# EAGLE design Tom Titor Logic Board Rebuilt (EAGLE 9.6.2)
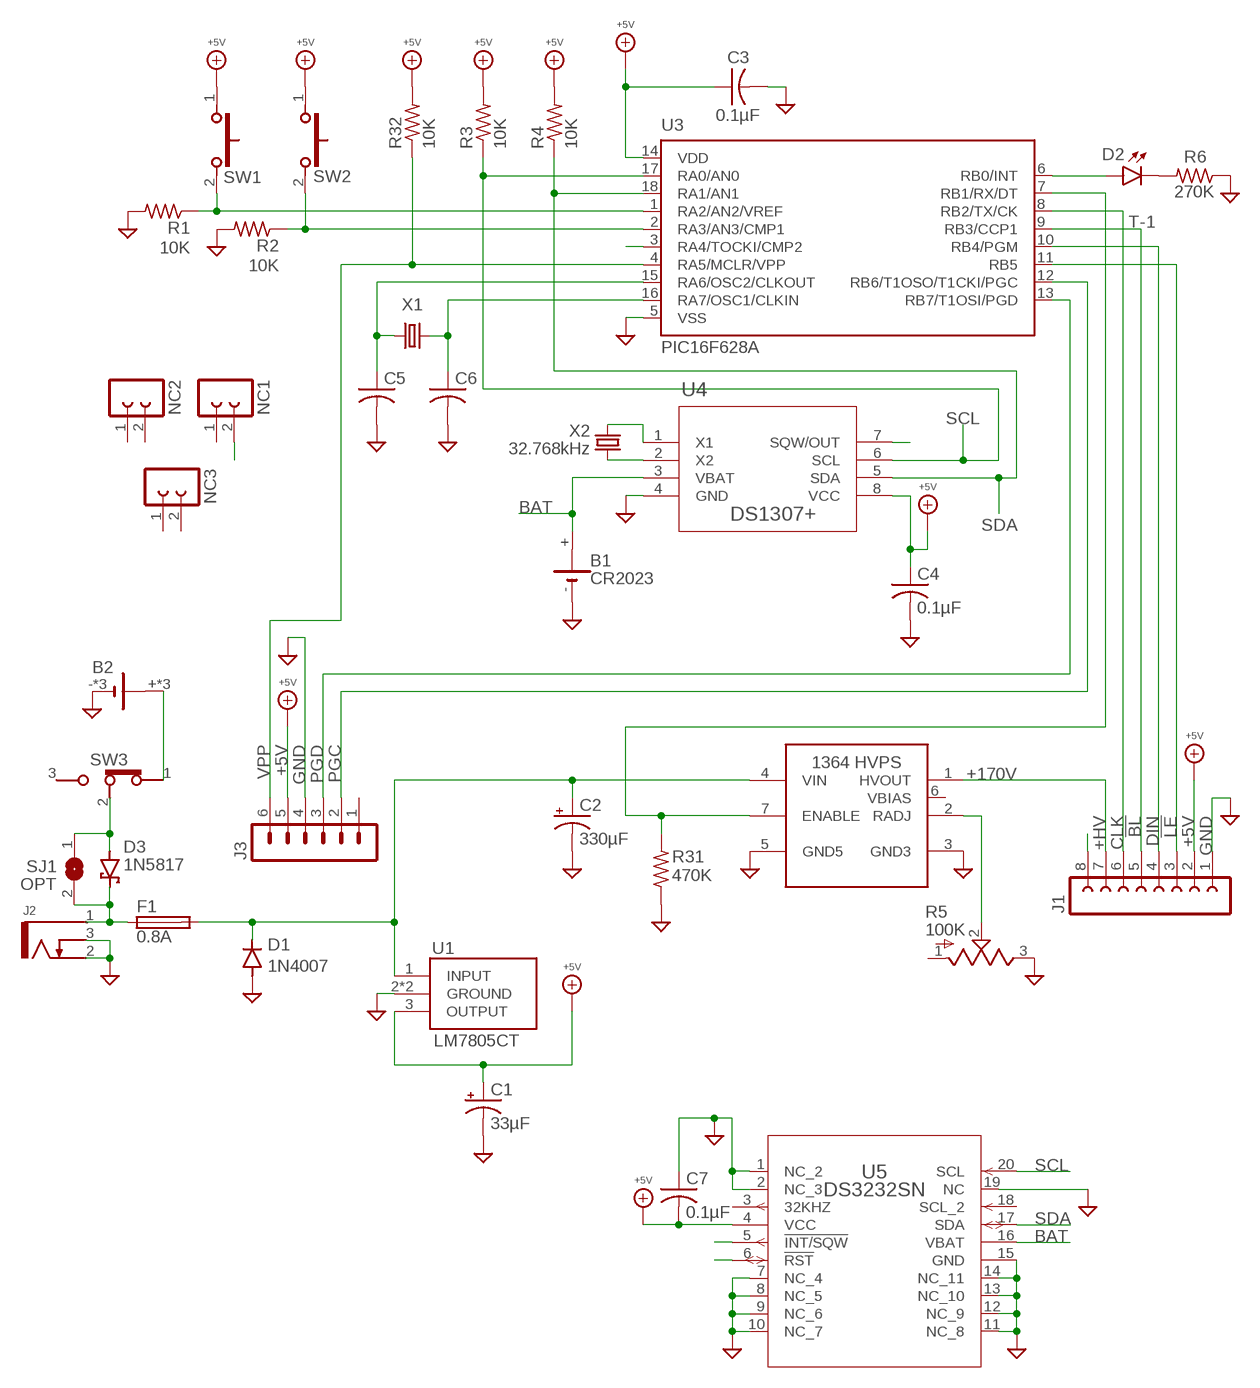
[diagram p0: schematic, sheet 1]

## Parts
B1  CR2023  BATTERY  [103]
B2  BATTERYWIRE_ATTACH  [BATTERY_WIRE]
C1  33µF  CPOL-USE2-5  [E2-5]
C2  330µF  CPOL-USE3.5-8  [E3,5-8]
C3  0.1µF  C-US  [C025-040X050]
C4  0.1µF  C-US  [C025-040X050]
C5  0.1µF  C-US  [C025-040X050]
C6  0.1µF  C-US  [C025-040X050]
C7  0.1µF  C-USC0805  [C0805]
D1  1N4007  RECTIFIER  [DO41-7]
D2  T-1  LED  [LED3MM]
D3  1N5817  SCHOTTKY  [DO41-7]
F1  0.8A  FUSE  [5X20MM]
J1  FE08  [FE08]
J2  KLDX-0202-B  [KDLX-0202-X]
J3  MA06  [MA06]
NC1  FE02  [FE02]
NC2  FE02  [FE02]
NC3  FE02  [FE02]
R1  10K  R-US0207/10  [0207/10]
R2  10K  R-US0207/10  [0207/10]
R3  10K  R-US0207/10  [0207/10]
R4  10K  R-US0207/10  [0207/10]
R5  100K  R-US_TRIM  [PV37W]
R6  270K  R-US0207/10  [0207/10]
R31  470K  R-US0207/10  [0207/10]
R32  10K  R-US0207/10  [0207/10]
SJ1  OPT  SJ  [SJ]
SW1  FSMRA4JH  SWITCH_PUSH_SPST_(ON)  [FSMRA4JH]
SW2  FSMRA4JH  SWITCH_PUSH_SPST_(ON)  [FSMRA4JH]
SW3  102-1261-EV  SWITCH_SLIDE_SPDT_ON  [SLIDE_SPDT_MINI]
U1  LM7805CT  MC7805CTG  [TO-220-3_RA]
U2  1364-HVPS-H  [1364-HVPS-H]
U3  PIC16F628A  PIC16F628P  [DIP-18]
U4  DS1307+  [DIP-8]
U5  DS3232SN  [SOIC-20]
X1  CRYSTAL  [HC18U-V_ALT]
X2  32.768kHz  CRYSTALTC38H  [TC38H]

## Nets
!BL!: J1.5 U3.9(RB3/CCP1)
!LE!: J1.3 U3.11(RB5)
+5V: C1.+ C3.1 C4.1 C7.2 J1.2 J3.5 R3.2 R4.2 R32.2 SW1.1 SW2.1 U1.3(OUTPUT) U3.14(VDD) U4.8(VCC) U5.4(VCC)
+9V: D3.C F1.1A F1.1B J2.1 SJ1.2
+9V_1: C2.+ D1.C F1.2A F1.2B U1.1(INPUT) U2.4(VIN)
+9V_2: D3.A SJ1.1 SW3.2(COM)
+9V_4: B2.+ B2.N$1(+) B2.N$2(+) SW3.1(POS_1)
+HV: J1.7 U2.1(HVOUT)
BAT: B1.+ U4.3(VBAT) U5.16(VBAT)
CLK: J1.6 U3.8(RB2/TX/CK)
DEBUG: D2.A D2.K(C) R6.2 U3.6(RB0/INT)
DIN: J1.4 U3.10(RB4/PGM)
ENABLE: R31.2 U2.7(ENABLE) U3.7(RB1/RX/DT)
GND: B1.- B2.- B2.N$3(-) B2.N$24(-) C1.- C2.- C3.2 C4.2 C5.2 C6.2 C7.1 D1.A J1.1 J2.2 J2.3 J3.4 R1.2 R2.2 R5.3 R6.1 R31.1 U1.2(GROUND) U1.2_1(GROUND) U2.3(GND3) U2.5(GND5) U3.5(VSS) U4.4(GND) U5.1(NC_2) U5.2(NC_3) U5.7(NC_4) U5.8(NC_5) U5.9(NC_6) U5.10(NC_7) U5.11(NC_8) U5.12(NC_9) U5.13(NC_10) U5.14(NC_11) U5.15(GND) U5.19(NC)
MYSTERY_1: J1.8
MYSTERY_2: U5.5(!INT/SQW)
MYSTERY_3: U5.6(!RST)
MYSTERY_4: U3.3(RA4/TOCKI/CMP2)
MYSTERY_5: U4.7(SQW/OUT)
N$1: U4.1(X1) X2.2
N$2: U4.2(X2) X2.1
N$5: NC1.2
PGC: J3.2 U3.12(RB6/T1OSO/T1CKI/PGC)
PGD: J3.3 U3.13(RB7/T1OSI/PGD)
RADJ: R5.2 U2.2(RADJ)
SCL: R3.1 U3.17(RA0/AN0) U4.6(SCL) U5.20(SCL)
SDA: R4.1 U3.18(RA1/AN1) U4.5(SDA) U5.17(SDA)
SUPP_CRYSTAL_1: C5.1 U3.15(RA6/OSC2/CLKOUT) X1.1
SUPP_CRYSTAL_2: C6.1 U3.16(RA7/OSC1/CLKIN) X1.2
SW1: R1.1 SW1.2 U3.1(RA2/AN2/VREF)
SW2: R2.1 SW2.2 U3.2(RA3/AN3/CMP1)
VPP: J3.6 R32.1 U3.4(RA5/MCLR/VPP)
Unconnected: J3.1 NC1.1 NC2.1 NC2.2 NC3.1 NC3.2 R5.1 SW3.3(POS_2) U2.6(VBIAS) U5.3(32KHZ) U5.18(SCL_2)

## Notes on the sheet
- +170V

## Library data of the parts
B1 B2 = My Imported Components:BATTERY: LI BATTERY Varta
C1 C2 = My Imported Components:CPOL-US
C3-C6 = My Imported Components:C-US
C7 = rcl:C-US: CAPACITOR, American symbol; SPICEPREFIX: C
D1 = My Imported Components:RECTIFIER
D2 = My Imported Components:LED
D3 = My Imported Components:SCHOTTKY
F1 = My Imported Components:FUSE
J1 = My Imported Components:FE08: FEMALE HEADER; OC_FARNELL: unknown; OC_NEWARK: unknown
J2 = My Imported Components:KLDX-0202-B: https://www.mouser.com/datasheet/2/222/KLDX_0202-334781.pdf
J3 = My Imported Components:MA06: PIN HEADER; OC_FARNELL: unknown; OC_NEWARK: unknown
NC1-NC3 = My Imported Components:FE02: FEMALE HEADER
R1-R4 R6 R31 R32 = My Imported Components:R-US: RESISTOR, American symbol; SPICEPREFIX: R
R5 = My Imported Components:R-US_TRIM: Res Cermet Trimmer 1M Ohm 10% 1/4W 12(Elec)Turn 1.8mm (6.4 X 4 X 7.7mm) Pin Thru-Hole Bulk Check prices; AVAILABILITY: Good; DESCRIPTION: 100 kOhms 0.25W, 1/4W PC Pins Through Hole Trimmer Potentiometer Cermet 12 Turn Top Adjustment; MF: Bourns; MP: PV37W104C01B00; PACKAGE: 3224X Bourns; PRICE: None; PURCHASE-URL: https://pricing.snapeda.com/search/part/PV37W104C01B00/?ref=eda
SJ1 = jumper:SJ: SMD solder JUMPER
SW1 SW2 = My Imported Components:SWITCH_PUSH_SPST_(ON)
SW3 = My Imported Components:SWITCH_SLIDE_SPDT_ON
U1 = My Imported Components:MC7805CTG: Voltage regulator,MC7805CT 5V 1A ON Semiconductor MC7805CTG, Single Linear Voltage Regulator, 1A 5 V, +/-4%, 3-Pin TO-220 Source: Datasheet; ARROW_PART_NUMBER: MC7805CTG; ARROW_PRICE-STOCK: https://www.arrow.com/en/products/mc7805ctg/on-semiconductor; DESCRIPTION: Voltage regulator,MC7805CT 5V 1A ON Semiconductor MC7805CTG, Single Linear Voltage Regulator, 1A 5 V, +/-4%, 3-Pin TO-220; HEIGHT: 4.82mm; MANUFACTURER_NAME: ON Semiconductor; MANUFACTURER_PART_NUMBER: MC7805CTG; MOUSER_PART_NUMBER: 863-MC7805CTG; MOUSER_PRICE-STOCK: https://www.mouser.co.uk/ProductDetail/ON-Semiconductor/MC7805CTG/?qs=%252B9%2Fcbd0IE0SRQQJXyw%252B9hQ%3D%3D
U2 = My Imported Components:1364-HVPS-H: https://www.shop-tes.com/content/Datasheets/8002K.pdf
U3 = My Imported Components:PIC16F62*: FLASH-Based 8-Bit CMOS Microcontroller Source: http://ww1.microchip.com/downloads/en/DeviceDoc/40300C.pdf; MF: MICROCHIP; MPN: PIC16F628-04I/P; OC_FARNELL: 9760407; OC_NEWARK: 19C7272
U4 = My Imported Components:DS1307+; BUILT_BY: EMA_UL_Team; MANUFACTURER_PART_NUMBER: DS1307+; SOURCELIBRARY: Maxim_2011-05-13; VENDOR: Maxim Integrated Products
U5 = My Imported Components:DS3232SN; BUILT_BY: EMA_UL_Team; MANUFACTURER_PART_NUMBER: ds3232sn#; SOURCELIBRARY: Maxim_2009-12-17_1; VENDOR: Maxim Integrated Products
X1 = My Imported Components:CRYSTAL
X2 = crystal:CRYSTAL: CRYSTAL; OC_FARNELL: unknown; OC_NEWARK: unknown

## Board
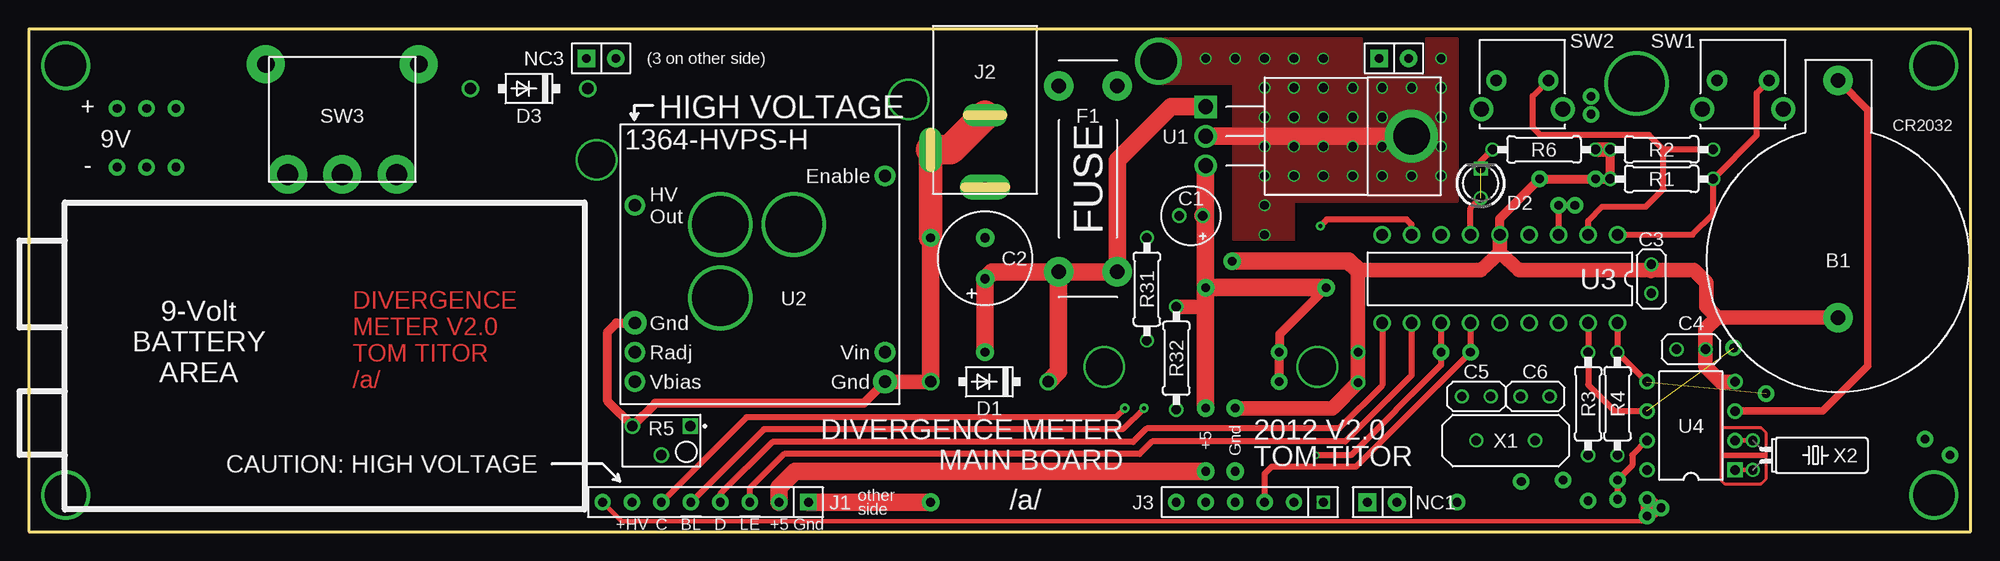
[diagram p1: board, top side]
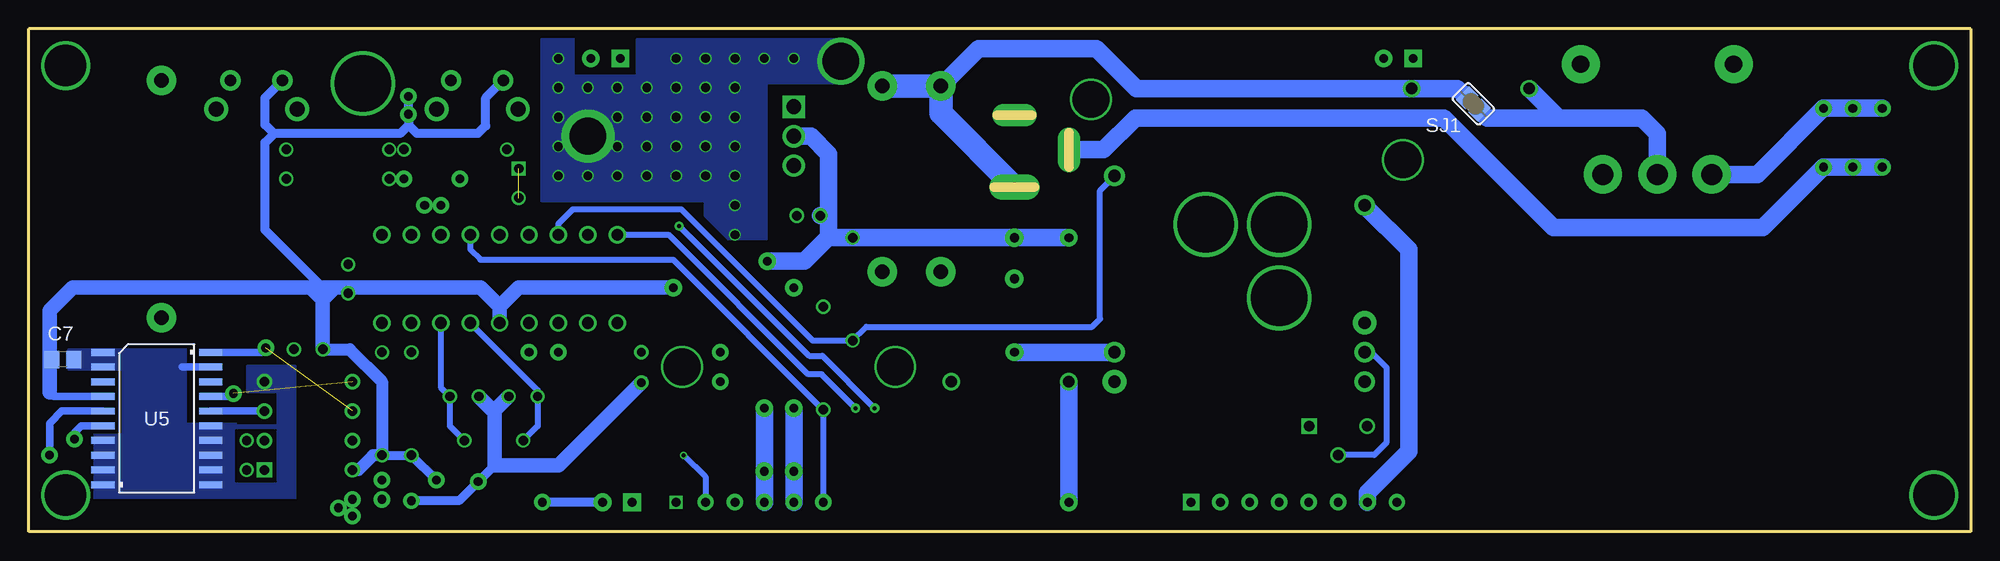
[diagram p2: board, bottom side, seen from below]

Size 167.64 x 43.43 mm. Coordinates in mm from the lower left corner, seen from the top.
Outline: 0,0 167.64,0 167.64,43.43 0,43.43 0,0
Copper layers (1*16): Top 0.035559375mm / dielectric 1.6mm / Bottom 0.035559375mm
Design rules "oshpark-2layer *": minimum track width 6mil, minimum drill 10mil, track to track 6mil, track to pad 6mil, pad to pad 6mil, via to via 6mil, smd to smd 6mil, copper to edge 15mil, drill to drill 6mil, minimum pad ring 5mil, minimum via ring 5mil, stop-mask expansion 2.5mil, vias tented up to drill 0mil, thermal gap 10mil

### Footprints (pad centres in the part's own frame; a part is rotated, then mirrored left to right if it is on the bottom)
103 = drill 1.27 pad 2.54: + 0,0; - 0,-20.498
BATTERY_WIRE = drill 0.75 pad 1.422: + 5.08,0; - 5.08,-5.08; N$1 0,0; N$2 2.54,0; N$3 0,-5.08; N$24 2.54,-5.08
E2-5 = drill 0.813 pad 1.27: + -1.016,0; - 1.016,0
E3,5-8 = drill 0.813 pad 1.6: + -1.778,0; - 1.778,0
C025-040X050 = drill 0.813: 1 -1.25,0; 2 1.25,0
C0805 = smd 1.3 x 1.5: 1 -0.95,0; 2 0.95,0
DO41-7 = drill 1: A 5.08,0; C -5.08,0
LED3MM = drill 0.813: A -1.27,0 | drill 0.813 square: K 1.27,0
5X20MM = drill 1.245 pad 2.54: 1A -8.026,2.54; 1B -8.026,-2.54; 2A 8.026,2.54; 2B 8.026,-2.54
FE08 = drill 0.75 pad 1.422 square: 1 -8.89,0 | drill 0.75 pad 1.422: 2 -6.35,0; 3 -3.81,0; 4 -1.27,0; 5 1.27,0; 6 3.81,0; 7 6.35,0; 8 8.89,0
KDLX-0202-X = drill 0.8 pad 2.184 long: 1 13.9,0 | drill 0.8 pad 1.93 long: 2 7.7,0; 3 10.7,-4.7
MA06 = drill 0.75 square: 1 -6.35,0 | drill 0.75 pad 1.422: 2 -3.81,0; 3 -1.27,0; 4 1.27,0; 5 3.81,0; 6 6.35,0
FE02 = drill 0.75 pad 1.524 square: 1 -1.27,0 | drill 0.75 pad 1.524: 2 1.27,0
0207/10 = drill 0.813: 1 -4.445,0; 2 4.445,0
PV37W = drill 0.9 square: 1 -2.5,-1.25 | drill 0.9: 2 0,1.25; 3 2.5,-1.25
SJ = smd 1.168 x 1.6: 1 -0.762,0; 2 0.762,0
FSMRA4JH = drill 0.991 pad 1.753: 1 4.496,0; 2 0,0 | drill 1.295 pad 2.057: 3 -1.245,2.489; 4 5.766,2.489
SLIDE_SPDT_MINI = drill 1.8 pad 3.302: 1 -4.699,0; 2 0,0; 3 4.699,0 | drill 1.5 pad 3.302: P$4 -6.604,9.525; P$5 6.604,9.525
TO-220-3_RA = drill 1.29 pad 1.935 square: 1 0,0 | drill 1.29 pad 1.935: 2 2.54,0; 3 5.08,0 | drill 3.175 pad 4.572: 2_1 2.54,17.78
1364-HVPS-H = drill 1.067 pad 1.778: 1 1.27,17.145; 2 1.27,4.445; 4 22.86,4.445; 6 1.27,1.905; 7 22.86,19.685 | drill 1.067 pad 2.032: 3 1.27,6.985; 5 22.86,1.905
DIP-18 = drill 1: 1 -10.16,-3.81; 2 -7.62,-3.81; 3 -5.08,-3.81; 4 -2.54,-3.81; 5 0,-3.81; 6 2.54,-3.81; 7 5.08,-3.81; 8 7.62,-3.81; 9 10.16,-3.81; 10 10.16,3.81; 11 7.62,3.81; 12 5.08,3.81; 13 2.54,3.81; 14 0,3.81; 15 -2.54,3.81; 16 -5.08,3.81; 17 -7.62,3.81; 18 -10.16,3.81
DIP-8 = drill 0.813 pad 1.321 square: 1 0,0 | drill 0.813 pad 1.321: 2 0,-2.54; 3 0,-5.08; 4 0,-7.62; 5 7.62,-7.62; 6 7.62,-5.08; 7 7.62,-2.54; 8 7.62,0
SOIC-20 = smd 2 x 0.6: 1 -4.65,5.715; 2 -4.65,4.445; 3 -4.65,3.175; 4 -4.65,1.905; 5 -4.65,0.635; 6 -4.65,-0.635; 7 -4.65,-1.905; 8 -4.65,-3.175; 9 -4.65,-4.445; 10 -4.65,-5.715; 11 4.65,-5.715; 12 4.65,-4.445; 13 4.65,-3.175; 14 4.65,-1.905; 15 4.65,-0.635; 16 4.65,0.635; 17 4.65,1.905; 18 4.65,3.175; 19 4.65,4.445; 20 4.65,5.715
HC18U-V_ALT = drill 0.813: 1 -2.54,0; 2 2.54,0
TC38H = drill 0.813: 1 -1.27,0; 2 1.27,0

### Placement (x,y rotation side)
B1  156.21,38.99 0 top
B2  7.62,36.58 0 top
C1  100.33,27.3 180 top
C2  82.55,23.62 90 top
C3  140.08,21.84 90 top
C4  143.51,15.75 0 top
C5  124.97,11.68 0 top
C6  130.05,11.68 180 top
C7  164.73,14.87 180 bottom
D1  82.93,12.95 180 top
D2  125.35,30.1 90 top
D3  43.18,38.28 180 top
F1  91.44,30.48 270 top
J1  58.42,2.54 180 top
J2  82.55,43.69 270 top
J3  105.41,2.54 180 top
NC1  116.84,2.54 0 top
NC2  117.86,40.89 0 top
NC3  49.4,40.89 0 top
R1  140.97,30.48 180 top
R2  140.97,33.02 180 top
R3  134.62,11.05 270 top
R4  137.16,11.05 270 top
R5  54.61,7.87 180 top
R6  130.81,33.02 180 top
R31  96.52,20.95 270 top
R32  99.06,14.99 90 top
SJ1  42.93,36.96 135 bottom
SW1  150.24,38.99 180 top
SW2  131.19,38.99 180 top
SW3  27.05,30.86 0 top
U1  101.6,36.7 270 top
U2  51.05,11.05 0 top
U3  127,21.84 180 top
U4  147.32,5.33 180 top
U5  156.6,9.78 0 bottom
X1  127.51,7.87 0 top
X2  148.84,6.6 270 top

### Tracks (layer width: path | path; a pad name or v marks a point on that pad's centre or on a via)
!BL!  (via drill 0.35 pad 0.79)
  Top 0.508: J1.5 63.45,8.84 94.44,8.84 v96.27,10.67
  Bottom 0.508: U3.9 112.42,25.65 100.36,13.59 99.19,13.59 v96.27,10.67
!LE!
  Top 0.508: U3.11 119.38,13.51 113.67,7.8 96.98,7.8 95.89,6.71 65.2,6.71 62.23,3.73 J1.3
+5V  (via drill 0.75 pad 1.42, 0.75 pad 1.52)
  Top 0.762: v112.01,21.08 107.97,17.04 v107.95,15.49 v107.95,12.95
  Top 1.27: R32.2 101.52,19.43 101.6,19.36
  Top 1.524: U1.3 101.6,27.3 | 101.6,27.3 v101.6,21.08 | v101.6,21.08 101.6,19.36 v101.6,10.67 | v101.6,5.21 66.17,5.21 64.77,3.81 J1.2 | v101.6,21.08 v112.01,21.08 | C1.+ 101.6,27.3
  Bottom 0.635: U5.4 165.48,11.68 165.84,12.04
  Bottom 0.762: R4.2 R3.2 v132.46,4.45 | 142.26,21.08 147.24,26.06 147.24,33.62 146.47,34.39 | 134.87,35.13 134.14,34.39 128.88,34.39 128.19,35.08 128.19,37.49 SW2.1 | 134.87,35.13 135.61,34.39 146.47,34.39 | 134.87,35.13 v134.87,36.07 v134.87,37.59 | 146.47,34.39 147.24,35.16 147.24,37.49 SW1.1
  Bottom 1.016: C4.1 139.93,15.75 137.16,12.98 R4.2 137.92,6.6 139.19,5.33 U4.8
  Bottom 1.27: 141.22,21.08 140.11,21.08 | 140.11,21.08 128.63,21.08 127,19.46 | v112.01,21.08 125.37,21.08 127,19.46 | C4.1 142.26,20.05 | 142.26,20.05 141.22,21.08 | C3.1 140.06,21.03 140.11,21.08 | 142.26,20.05 143.3,21.08 | 141.22,21.08 142.26,21.08 143.3,21.08 | U3.14 127,19.46 | 165.84,12.04 165.84,14.96 | 165.84,14.96 165.84,19.13 163.88,21.08 143.3,21.08 | C7.2 165.69,14.96 165.84,14.96
  Bottom 1.524: v101.6,10.67 v101.6,5.21 J3.5
+9V
  Bottom 1.016: 43.71,37.69 43.49,37.47 SJ1.2
  Bottom 1.524: F1.1B 85.67,41.73 75.49,41.73 72.03,38.28 D3.C 44.3,38.28 43.71,37.69
  Bottom 2.032: J2.1 88.9,36.14 F1.1B F1.1A
+9V_1  (via drill 0.75 pad 1.52)
  Top 1.524: F1.2B F1.2A 93.98,32.08 98.6,36.7 U1.1 | F1.2B 83.16,22.45 C2.+ v82.55,15.49 | F1.2B 88.9,13.84 D1.C
  Bottom 1.524: U2.4 v82.55,15.49
+9V_2
  Bottom 1.016: SJ1.1 42.41,36.39 42.11,36.09
  Bottom 1.524: SW3.2 27.05,34.39 28.37,35.71 35.53,35.71 | D3.A 35.53,35.71 | 42.11,36.09 41.73,35.71 35.53,35.71
+9V_4
  Bottom 1.524: SW3.1 18.41,30.86 B2.+ B2.N$2 B2.N$1
+HV
  Bottom 1.524: U2.1 48.51,24.38 48.51,6.93 52.07,3.38 J1.7
BAT
  Top 0.635: U4.3 154.86,10.41 158.78,14.33 158.78,36.42 B1.+
  Bottom 0.635: U4.3 U5.16
CLK  (via drill 0.35 pad 0.79)
  Top 0.508: U3.8 119.38,26.54 118.95,26.98 112.06,26.98 v111.51,26.42 | v94.61,10.67 93.83,9.88 61.95,9.88 J1.6
  Bottom 0.508: v111.51,26.42 100.28,15.19 99.14,15.19 v94.61,10.67
DEBUG  (1 unrouted)
  Top 0.508: U3.6 124.46,27.94 D2.A | D2.K 125.35,32 R6.2
DIN
  Top 0.508: U3.10 116.84,12.65 113.11,8.91 96.5,8.91 95.33,7.75 64.19,7.75 59.69,3.25 J1.4
ENABLE
  Bottom 0.508: U2.7 75.16,29.49 75.16,18.39 75.84,17.7 95.33,17.7 R31.2 99.97,16.51 111.33,27.86 120.67,27.86 121.92,26.62 U3.7
GND  (via drill 0.75, 0.75 pad 1.27, 0.75 pad 1.42, 0.75 pad 1.52, 3.17 pad 4.06)
  Top 0.254: 146.08,12.95 146.08,8.97 | 149.99,6.53 149.99,4.57 149.56,4.14 146.39,4.14 146.08,4.45 146.08,6.53 | 149.99,6.53 149.99,6.73 | 149.99,6.73 149.99,8.53 149.56,8.97 146.08,8.97 | 146.08,8.97 146.08,6.73 | 146.08,6.73 146.08,6.53 | 146.08,6.73 149.99,6.73 | 146.08,6.53 149.99,6.53
  Top 0.762: U2.5 72.06,11.1 54.09,11.1 R5.3 49.96,11.27 49.96,17.27 50.72,18.03 U2.3 | U3.5 127,27.05 v130.43,30.48 v135.25,30.48 R1.2 R2.2
  Top 1.27: D1.A U2.5 | 140.03,22.61 128.63,22.61 127,24.13 | 140.03,22.61 143.74,22.61 144.83,21.51 144.83,19.46 145.77,18.52 | C3.2 140.06,22.53 140.03,22.61 | U3.5 127,24.13 | 127,24.13 125.37,22.61 114.76,22.61 v114.76,15.49 v114.76,12.88 112.55,10.67 v104.14,10.67 | B1.- 145.77,18.52 | 145.77,18.52 144.76,17.51 C4.2 144.76,14.28 146.08,12.95 U4.4 | R6.1 R2.2
  Top 1.524: v77.85,25.4 D1.A | J1.1 v77.85,2.54 | v103.89,23.37 113.94,23.37 114.76,22.61 | U1.2 U1.2_1
  Top 2.032: J2.3 v77.85,25.4
  Top 2.54: J2.2 79.55,32.99 J2.3
  Bottom 0.635: U5.19 154.41,14.22
  Bottom 0.762: 127.43,5.74 v128.85,4.32 130.5,2.67 v134.62,2.67
  Bottom 1.27: v114.76,12.88 121.89,5.74 127.43,5.74 127.43,10.32 | C6.2 127.43,10.32 | C5.2 127.43,10.47 127.43,10.32
  Bottom 1.524: v77.85,25.4 C2.- R31.1 98.6,25.4 | D1.A v77.85,2.54 | 98.6,25.4 98.6,27.3 | 98.6,27.3 98.6,32.64 100.13,34.16 U1.2 | 98.6,25.4 98.65,25.4 100.69,23.37 v103.89,23.37 | v104.14,10.67 v104.14,5.21 J3.4 | J2.3 74.86,32.99 72.11,35.74 45.49,35.74 36.02,26.26 17.93,26.26 B2.- B2.N$24 B2.N$3 | C1.- 98.6,27.3
  other vias: 101.6,40.89 104.14,40.89 106.68,40.89 109.22,40.89 111.76,40.89 106.68,38.35 109.22,38.35 111.76,38.35 114.3,38.35 97.54,40.64 116.84,38.35 119.38,38.35 121.92,38.35 121.92,35.81 121.92,33.27 121.92,30.73 119.38,30.73 116.84,30.73 114.3,30.73 111.76,30.73 109.22,30.73 106.68,30.73 106.68,28.19 106.68,25.65 106.68,33.27 109.22,33.27 111.76,33.27 114.3,33.27 116.84,33.27 116.84,35.81 114.3,35.81 111.76,35.81 109.22,35.81 106.68,35.81 121.92,40.89
  pour Top (no thermals): 97.61,42.6 97.61,38.68 103.96,38.68 103.96,25.22 109.27,25.22 109.27,28.52 123.37,28.52 123.37,42.6 120.6,42.6 120.6,39.42 115.11,39.42 115.11,42.6
  pour Bottom (no thermals): 97.61,42.6 97.61,38.68 103.96,38.68 103.96,25.22 107.26,25.22 109.27,27.23 109.27,28.52 123.37,28.52 123.37,42.6 120.6,42.6 120.6,39.42 115.11,39.42 115.11,42.6
  pour Bottom (no thermals): 146.18,12.01 148.79,12.01 148.79,14.35 144.65,14.35 144.65,2.87 161.98,2.87 161.98,8.41 159.54,8.41 159.54,13.97 164.19,13.97 164.19,15.8 154.13,15.8 154.13,9.37 149.78,9.37 149.78,9.22 146.18,9.22
  cutout Bottom (no thermals): 146.33,8.76 149.78,8.76 149.78,4.34 146.33,4.34
MYSTERY_1  (via drill 0.75 pad 1.42)
  Top 0.381: J1.8 51.16,0.91 139.27,0.91 v139.7,1.35
  Top 1.016: v139.7,1.35 v139.7,2.79 v140.92,2.06 v139.7,1.35
MYSTERY_2  (via drill 0.75 pad 1.42)
  Bottom 0.635: v165.86,6.6 165.86,9.35 164.79,10.41 U5.5
MYSTERY_3  (via drill 0.75 pad 1.42)
  Bottom 0.635: v163.7,8 163.7,8.56 163.12,9.14 U5.6
MYSTERY_4  (via drill 0.75 pad 1.42)
  Top 0.508: U3.3 v132.08,28.19 v133.48,28.19
MYSTERY_5  (via drill 0.75 pad 1.42)
  Top 0.508: U4.7 138.43,6.6 138.43,5.71 v137.16,4.45 v137.16,2.79
N$1
  Top 0.381: X2.2 U4.1
N$2
  Top 0.381: X2.1 U4.2
N$3  (via drill 3.17 pad 3.61)
  other vias: 49.02,32.13
N$5  (via drill 0.75 pad 1.42)
  Bottom 0.762: NC1.2 v123.32,2.54
N$21  (via drill 3.58 pad 4.27)
  other vias: 3.17,40.26
N$22  (via drill 3.58 pad 4.27)
  other vias: 3.17,3.17
N$23  (via drill 3.58 pad 4.27)
  other vias: 164.47,40.26
N$24  (via drill 3.58 pad 4.27)
  other vias: 164.47,3.17
N$25  (via drill 3.17 pad 3.61)
  other vias: 75.95,37.34
N$26  (via drill 3.17 pad 3.61)
  other vias: 92.84,14.22
N$27  (via drill 3.17 pad 3.61)
  other vias: 111.25,14.22
N$28  (via drill 4.88 pad 5.59)
  other vias: 59.69,26.54
N$29  (via drill 4.88 pad 5.59)
  other vias: 66.04,26.54
N$30  (via drill 4.88 pad 5.59)
  other vias: 59.69,20.19
N$31  (via drill 4.88 pad 5.59)
  other vias: 138.81,38.73
PGC  (via drill 0.35, 0.75 pad 1.42)
  Top 0.508: U3.12 v121.92,15.49 121.92,14.4 114.12,6.6 v111.12,6.6
  Bottom 0.508: v111.12,6.6 109.22,4.75 J3.2
PGD  (via drill 0.75 pad 1.42)
  Top 0.508: U3.13 v124.46,15.49 114.58,5.61 107.29,5.61 106.68,5 J3.3
RADJ
  Bottom 0.508: R5.2 51.49,6.62 50.39,7.72 50.39,14.15 51.74,15.49 U2.2
SCL  (via drill 0.75 pad 1.42)  (1 unrouted)
  Top 0.508: U3.17 R3.1 134.62,12.7 136.91,10.41 U4.6
  Bottom 0.635: U5.20 147.57,15.49 v147.19,15.88
SDA  (via drill 0.75 pad 1.42)  (1 unrouted)
  Top 0.508: U3.18 R4.1 U4.5
  Bottom 0.635: v149.99,11.94 150.24,11.68 U5.17
SUPP_CRYSTAL_1
  Bottom 0.508: U3.15 123.72,12.21 C5.1 123.72,9.12 X1.1
SUPP_CRYSTAL_2
  Bottom 0.508: U3.16 132.08,12.47 C6.1 131.3,9.12 X1.2
SW1
  Top 0.508: U3.1 143.64,25.65 145.41,27.43 R1.1 149.17,34.24 149.17,37.92 SW1.2
SW2
  Top 0.508: U3.2 134.62,26.87 135.81,28.07 139.6,28.07 141.12,29.59 141.12,33.02 | 141.12,33.02 139.88,34.27 130.5,34.27 129.84,34.92 129.84,37.64 SW2.2 | R2.1 141.12,33.02
VPP
  Bottom 0.508: J3.6 R32.1 112.01,23.5 128.65,23.5 129.54,24.38 U3.4

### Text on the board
Top: DIVERGENCE / METER V2.0 / TOM TITOR / /a/
tPlace: (3 on other side) | + | HIGH VOLTAGE | CR2032 | 9V | - | 9-Volt / BATTERY / AREA | DIVERGENCE METER / MAIN BOARD | 2012 V2.0 / TOM TITOR | +5 | Gnd | CAUTION: HIGH VOLTAGE | /a/ | other / side | +HV | C | !BL! | D | !LE! | +5 | Gnd
tStop: DIVERGENCE / METER V2.0 / TOM TITOR / /a/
